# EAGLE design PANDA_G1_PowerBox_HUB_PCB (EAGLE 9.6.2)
BOARD_NAME: PwrBoxHUB

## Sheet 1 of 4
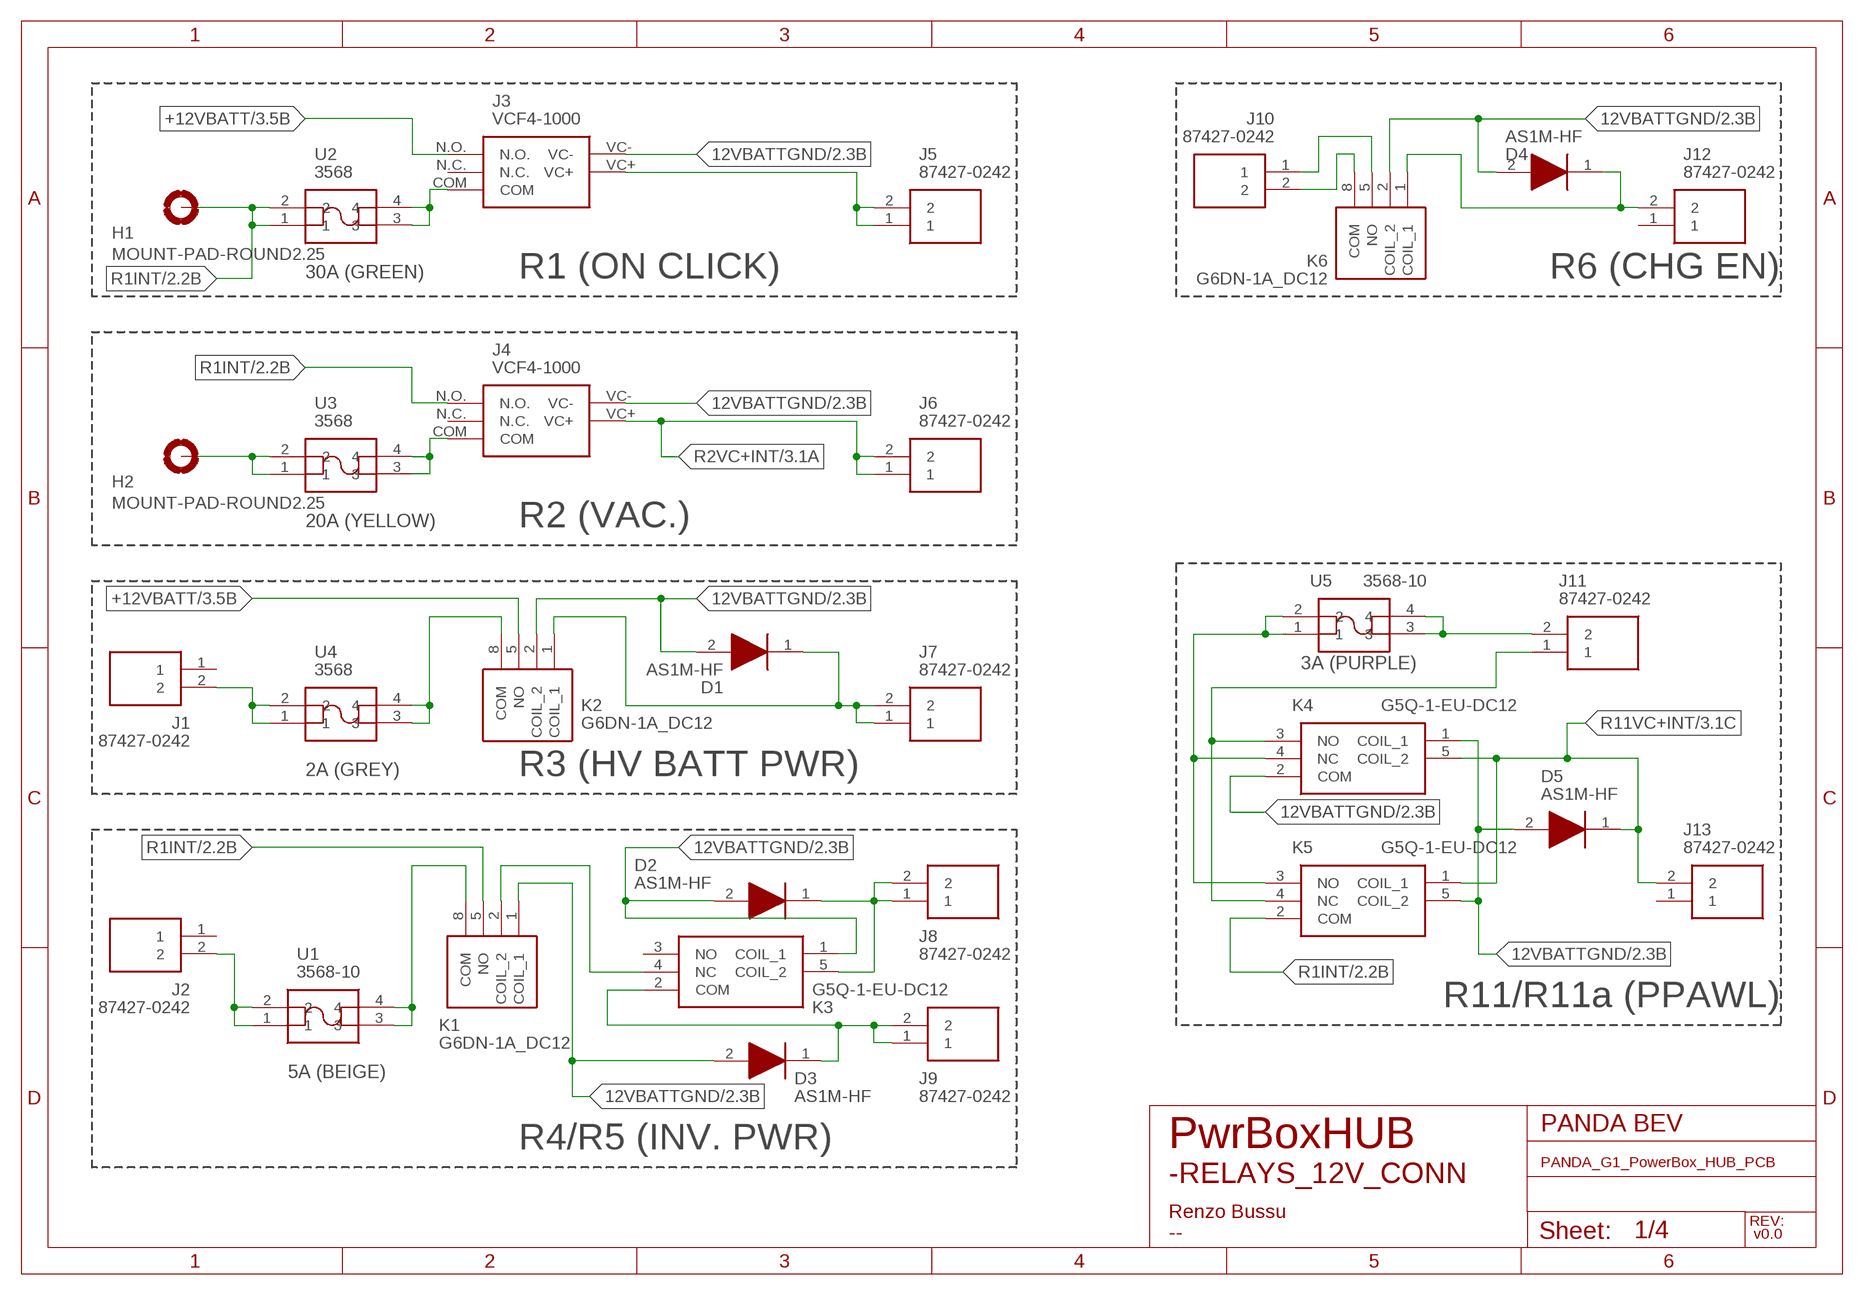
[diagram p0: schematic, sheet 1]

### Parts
D1  AS1M-HF  [DIOM5126X215N]
D2  AS1M-HF  [DIOM5126X215N]
D3  AS1M-HF  [DIOM5126X215N]
D4  AS1M-HF  [DIOM5126X215N]
D5  AS1M-HF  [DIOM5126X215N]
H1  MOUNT-PAD-ROUND2.25  [2,25-PAD]
H2  MOUNT-PAD-ROUND2.25  [2,25-PAD]
J1  87427-0242  [874270242]
J2  87427-0242  [874270242]
J3  VCF4-1000  [VCF4-1000]
J4  VCF4-1000  [VCF4-1000]
J5  87427-0242  [874270242]
J6  87427-0242  [874270242]
J7  87427-0242  [874270242]
J8  87427-0242  [874270242]
J9  87427-0242  [874270242]
J10  87427-0242  [874270242]
J11  87427-0242  [874270242]
J12  87427-0242  [874270242]
J13  87427-0242  [874270242]
K1  G6DN-1A_DC12  [G6DN1ADC12]
K2  G6DN-1A_DC12  [G6DN1ADC12]
K3  G5Q-1-EU-DC12  [G5Q1EUDC12]
K4  G5Q-1-EU-DC12  [G5Q1EUDC12]
K5  G5Q-1-EU-DC12  [G5Q1EUDC12]
K6  G6DN-1A_DC12  [G6DN1ADC12]
U1  3568-10  [356810]
U2  3568  [3568]
U3  3568  [3568]
U4  3568  [3568]
U5  3568-10  [356810]

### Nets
12VBATTGND: D1.2(A) D2.2(A) D3.2(A) D4.2(A) D5.2(A) J3.VC- J4.VC- K1.1(COIL_1) K2.2(COIL_2) K3.1(COIL_1) K4.1(COIL_1) K4.2(COM) K5.5(COIL_2) K6.2(COIL_2) ; also sheet 2,3,4
+12VBATT: J3.N.O. K2.5(NO) ; also sheet 3,4
N$2: J3.COM U2.3 U2.4
N$3: J4.COM U3.3 U3.4
N$4: J3.VC+ J5.1 J5.2
N$5: H2.B2,25(MOUNT) U3.1 U3.2
N$6: K2.8(COM) U4.3 U4.4
N$7: J1.2 U4.1 U4.2
N$8: D1.1(K) J7.1 J7.2 K2.1(COIL_1)
N$9: J2.2 U1.1 U1.2
N$10: K1.8(COM) U1.3 U1.4
N$11: D2.1(K) J8.1 J8.2 K3.5(COIL_2)
N$12: D3.1(K) J9.1 J9.2 K3.2(COM)
N$13: K1.2(COIL_2) K3.4(NC)
N$14: J10.2 K6.8(COM)
N$15: J10.1 K6.5(NO)
N$16: D4.1(K) J12.2 K6.1(COIL_1)
N$27: J11.2 U5.3 U5.4
N$28: K4.4(NC) K5.3(NO) U5.1 U5.2
N$30: J11.1 K4.3(NO) K5.4(NC)
R1INT: H1.B2,25(MOUNT) J4.N.O. K1.5(NO) K5.2(COM) U2.1 U2.2 ; also sheet 2,4
R2VC+INT: J4.VC+ J6.1 J6.2 ; also sheet 3
R11VC+INT: D5.1(K) J13.2 K4.5(COIL_2) K5.1(COIL_1) ; also sheet 3
Unconnected: J1.1 J2.1 J3.N.C. J4.N.C. J12.1 J13.1 K3.3(NO)

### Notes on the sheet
- 30A (GREEN) | R1 (ON CLICK) | R6 (CHG EN)
- 20A (YELLOW) | R2 (VAC.)
- 3A (PURPLE)
- 2A (GREY) | R3 (HV BATT PWR)
- R11/R11a (PPAWL)
- 5A (BEIGE)
- R4/R5 (INV. PWR)
- -RELAYS_12V_CONN
- Renzo Bussu
- v0.0
- --

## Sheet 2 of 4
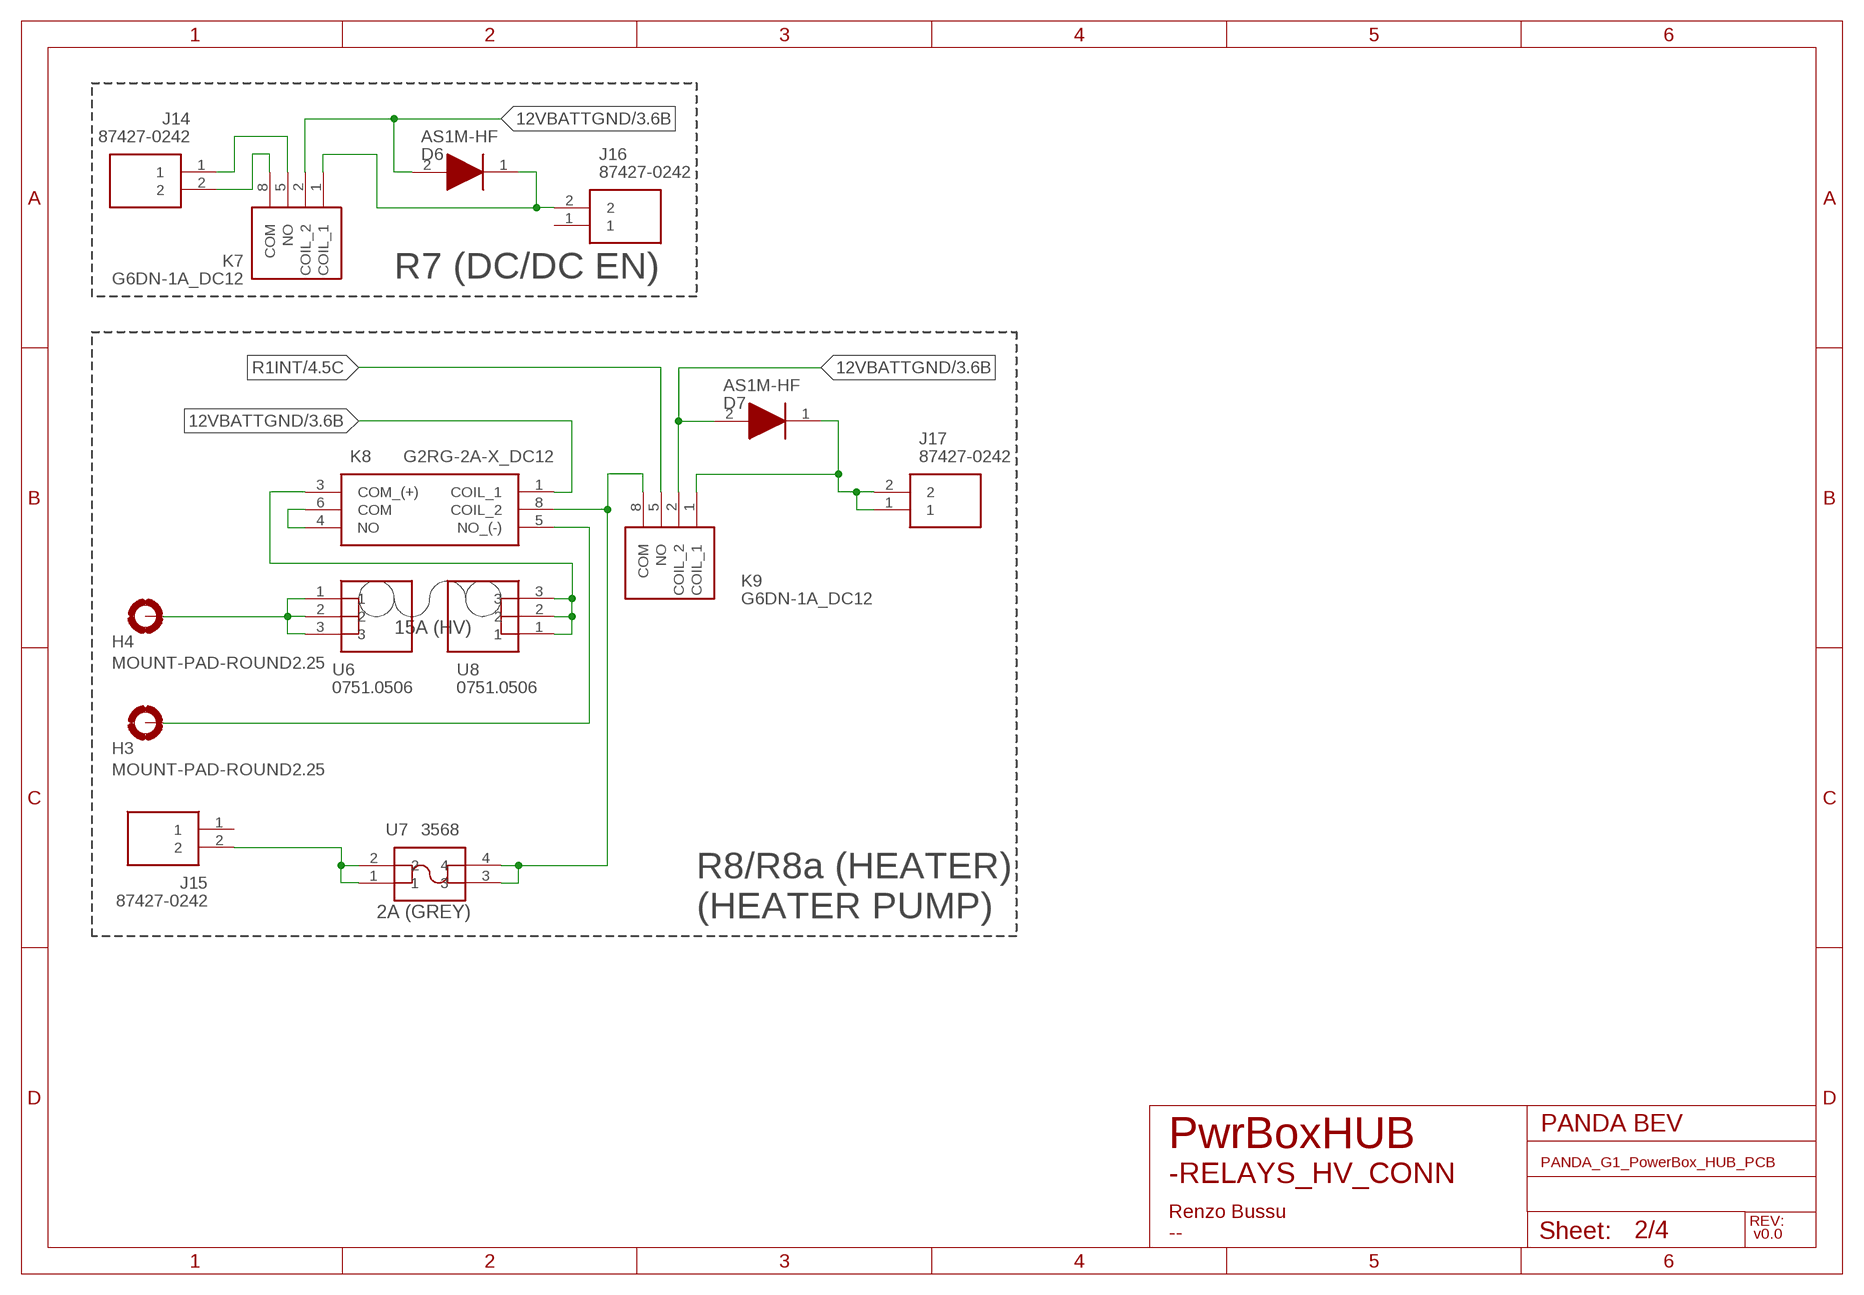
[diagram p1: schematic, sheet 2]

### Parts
D6  AS1M-HF  [DIOM5126X215N]
D7  AS1M-HF  [DIOM5126X215N]
H3  MOUNT-PAD-ROUND2.25  [2,25-PAD]
H4  MOUNT-PAD-ROUND2.25  [2,25-PAD]
J14  87427-0242  [874270242]
J15  87427-0242  [874270242]
J16  87427-0242  [874270242]
J17  87427-0242  [874270242]
K7  G6DN-1A_DC12  [G6DN1ADC12]
K8  G2RG-2A-X_DC12  [G2RG2AXDC12]
K9  G6DN-1A_DC12  [G6DN1ADC12]
U6  0751.0506  [07510506]
U7  3568  [3568]
U8  0751.0506  [07510506]

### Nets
12VBATTGND: D6.2(A) D7.2(A) K7.2(COIL_2) K8.1(COIL_1) K9.2(COIL_2) ; also sheet 1,3,4
N$17: J14.2 K7.8(COM)
N$18: J14.1 K7.5(NO)
N$19: D6.1(K) J16.2 K7.1(COIL_1)
N$20: H3.B2,25(MOUNT) K8.5(NO_(-))
N$21: K8.4(NO) K8.6(COM)
N$22: K8.3(COM_(+)) U8.1 U8.2 U8.3
N$23: D7.1(K) J17.1 J17.2 K9.1(COIL_1)
N$24: H4.B2,25(MOUNT) U6.1 U6.2 U6.3
N$25: K8.8(COIL_2) K9.8(COM) U7.3 U7.4
N$26: J15.2 U7.1 U7.2
R1INT: K9.5(NO) ; also sheet 1,4
Unconnected: J15.1 J16.1

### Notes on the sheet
- R7 (DC/DC EN)
- 15A (HV)
- 2A (GREY)
- R8/R8a (HEATER)
  (HEATER PUMP)
- -RELAYS_HV_CONN
- Renzo Bussu
- v0.0
- --

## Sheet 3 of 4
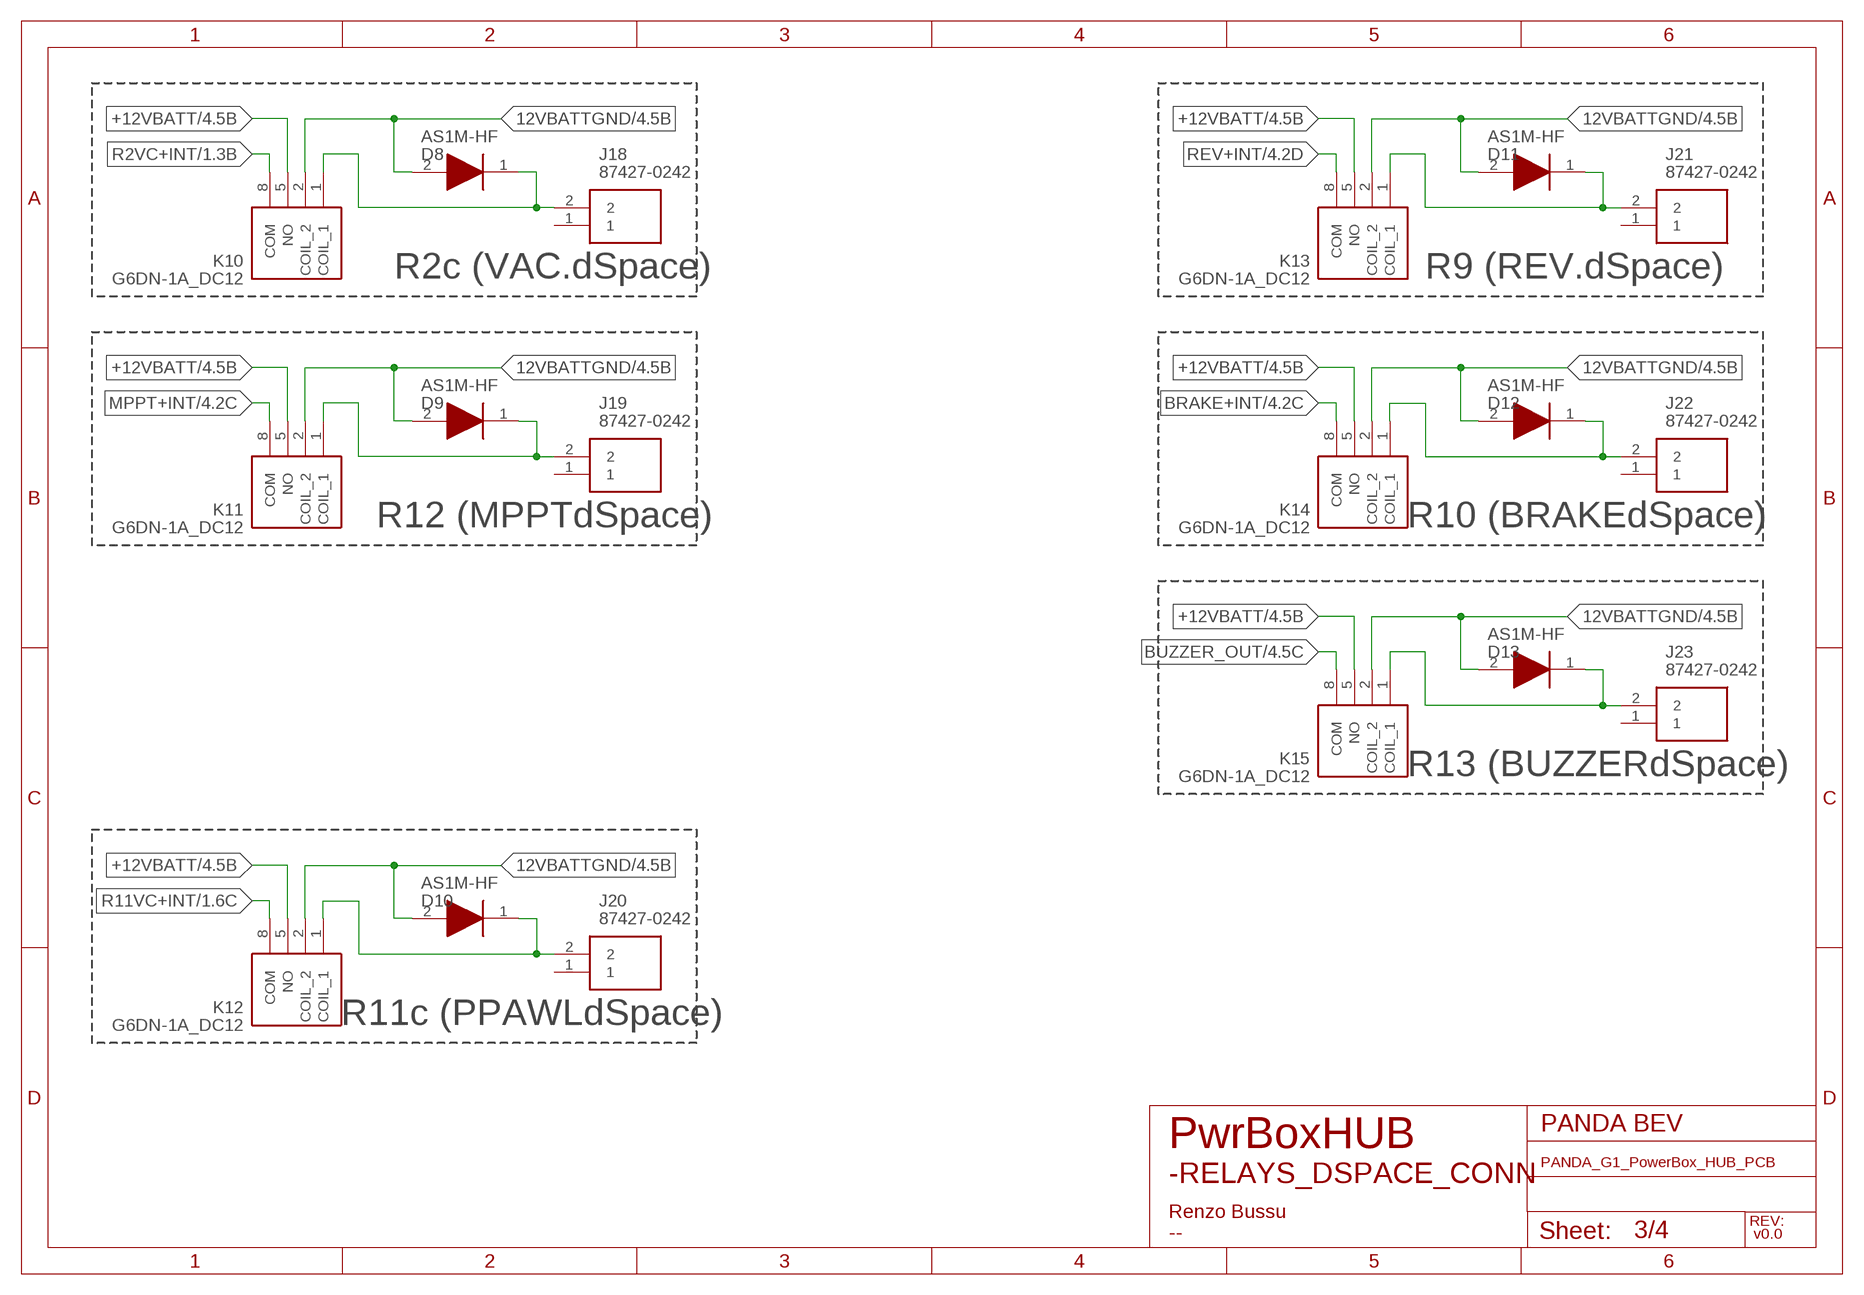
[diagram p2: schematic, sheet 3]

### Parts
D8  AS1M-HF  [DIOM5126X215N]
D9  AS1M-HF  [DIOM5126X215N]
D10  AS1M-HF  [DIOM5126X215N]
D11  AS1M-HF  [DIOM5126X215N]
D12  AS1M-HF  [DIOM5126X215N]
D13  AS1M-HF  [DIOM5126X215N]
J18  87427-0242  [874270242]
J19  87427-0242  [874270242]
J20  87427-0242  [874270242]
J21  87427-0242  [874270242]
J22  87427-0242  [874270242]
J23  87427-0242  [874270242]
K10  G6DN-1A_DC12  [G6DN1ADC12]
K11  G6DN-1A_DC12  [G6DN1ADC12]
K12  G6DN-1A_DC12  [G6DN1ADC12]
K13  G6DN-1A_DC12  [G6DN1ADC12]
K14  G6DN-1A_DC12  [G6DN1ADC12]
K15  G6DN-1A_DC12  [G6DN1ADC12]

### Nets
12VBATTGND: D8.2(A) D9.2(A) D10.2(A) D11.2(A) D12.2(A) D13.2(A) K10.2(COIL_2) K11.2(COIL_2) K12.2(COIL_2) K13.2(COIL_2) K14.2(COIL_2) K15.2(COIL_2) ; also sheet 1,2,4
+12VBATT: K10.5(NO) K11.5(NO) K12.5(NO) K13.5(NO) K14.5(NO) K15.5(NO) ; also sheet 1,4
BRAKE+INT: K14.8(COM) ; also sheet 4
BUZZER_OUT: K15.8(COM) ; also sheet 4
MPPT+INT: K11.8(COM) ; also sheet 4
N$32: D8.1(K) J18.2 K10.1(COIL_1)
N$33: D10.1(K) J20.2 K12.1(COIL_1)
N$36: D11.1(K) J21.2 K13.1(COIL_1)
N$37: D12.1(K) J22.2 K14.1(COIL_1)
N$38: D13.1(K) J23.2 K15.1(COIL_1)
N$39: D9.1(K) J19.2 K11.1(COIL_1)
R2VC+INT: K10.8(COM) ; also sheet 1
R11VC+INT: K12.8(COM) ; also sheet 1
REV+INT: K13.8(COM) ; also sheet 4
Unconnected: J18.1 J19.1 J20.1 J21.1 J22.1 J23.1

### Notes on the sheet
- R2c (VAC.dSpace) | R9 (REV.dSpace)
- R12 (MPPTdSpace) | R10 (BRAKEdSpace)
- R13 (BUZZERdSpace)
- R11c (PPAWLdSpace)
- -RELAYS_DSPACE_CONN
- Renzo Bussu
- v0.0
- --

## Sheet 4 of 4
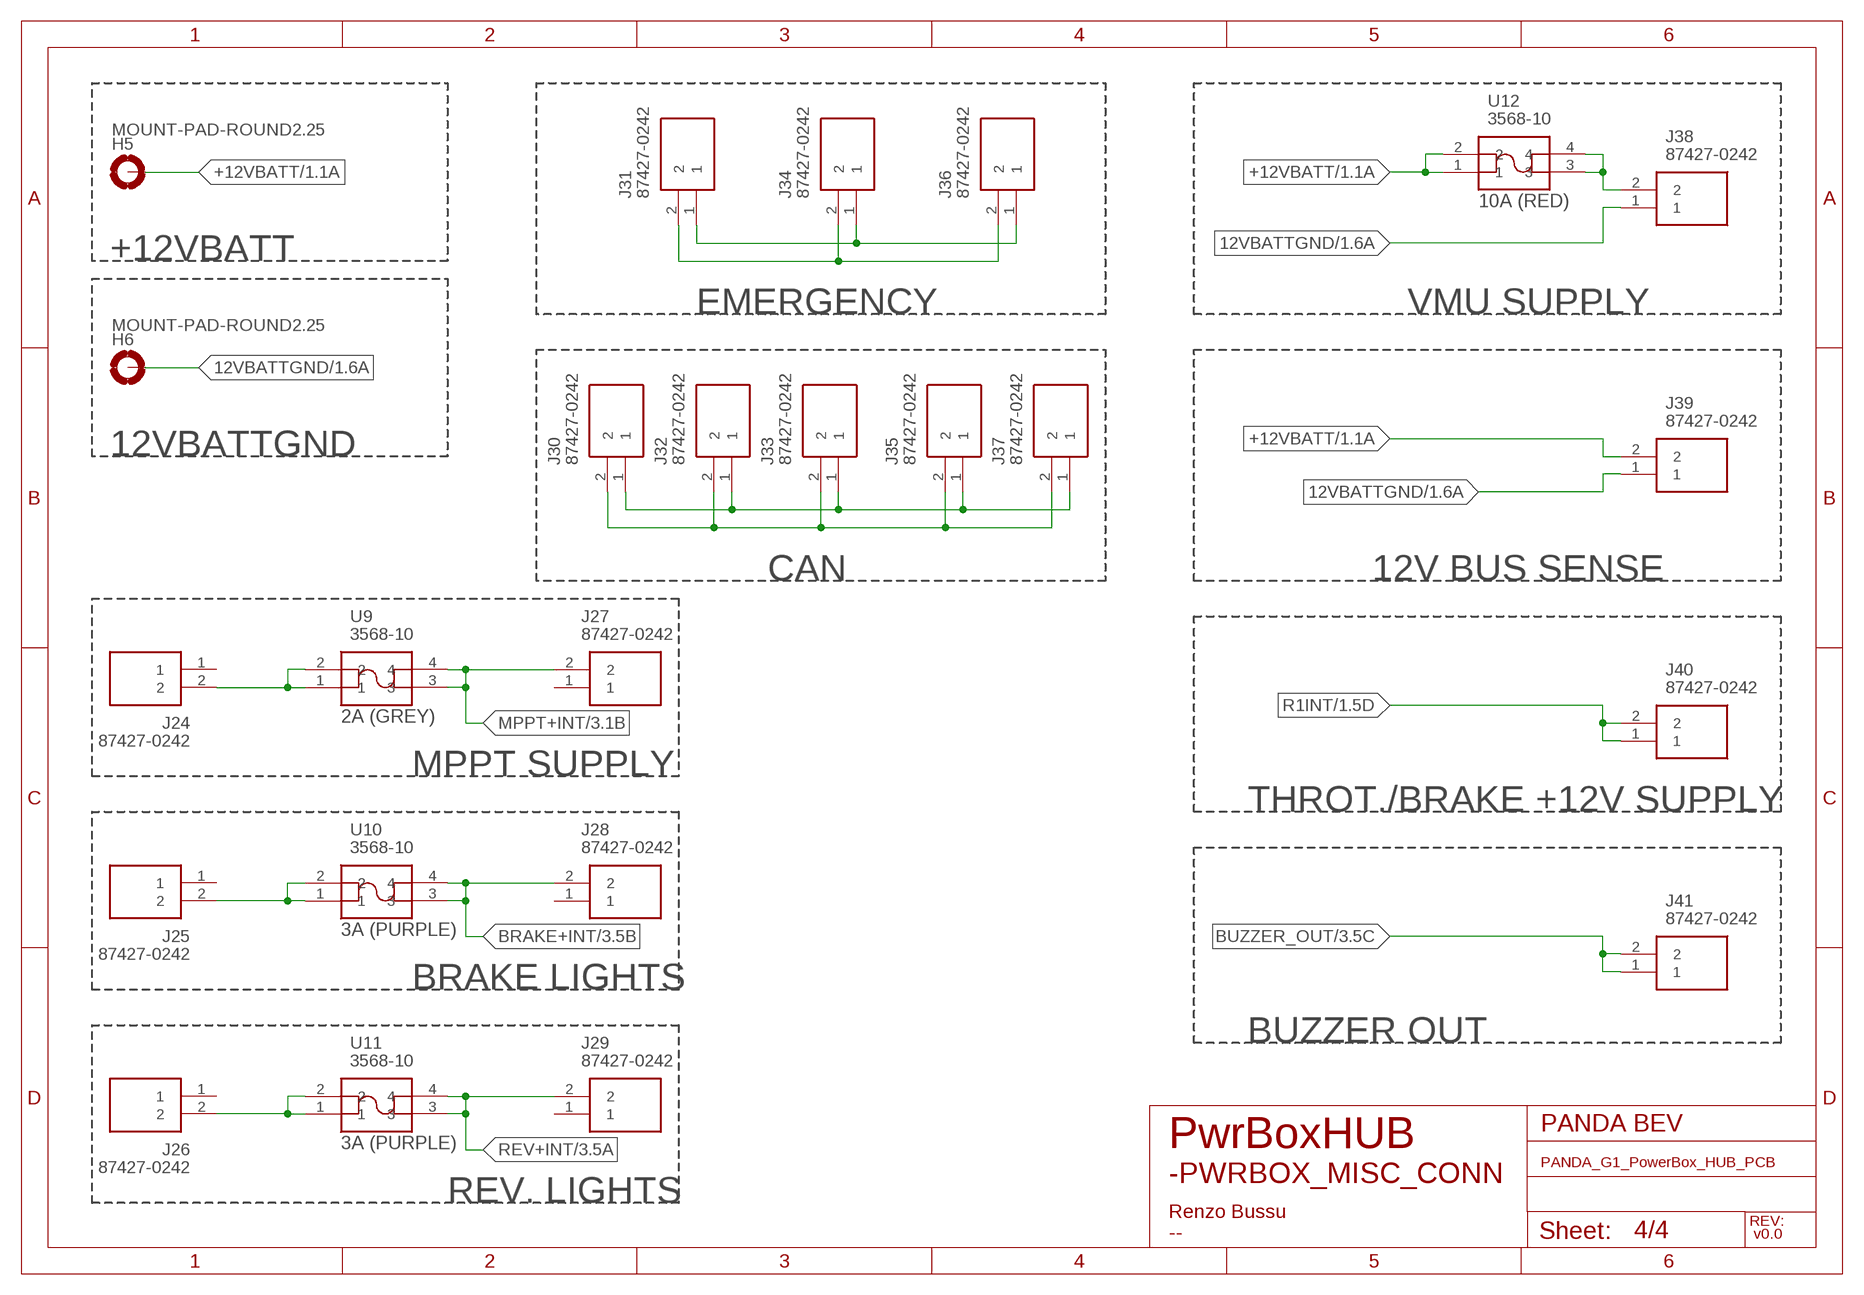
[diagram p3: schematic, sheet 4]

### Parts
H5  MOUNT-PAD-ROUND2.25  [2,25-PAD]
H6  MOUNT-PAD-ROUND2.25  [2,25-PAD]
J24  87427-0242  [874270242]
J25  87427-0242  [874270242]
J26  87427-0242  [874270242]
J27  87427-0242  [874270242]
J28  87427-0242  [874270242]
J29  87427-0242  [874270242]
J30  87427-0242  [874270242]
J31  87427-0242  [874270242]
J32  87427-0242  [874270242]
J33  87427-0242  [874270242]
J34  87427-0242  [874270242]
J35  87427-0242  [874270242]
J36  87427-0242  [874270242]
J37  87427-0242  [874270242]
J38  87427-0242  [874270242]
J39  87427-0242  [874270242]
J40  87427-0242  [874270242]
J41  87427-0242  [874270242]
U9  3568-10  [356810]
U10  3568-10  [356810]
U11  3568-10  [356810]
U12  3568-10  [356810]

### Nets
12VBATTGND: H6.B2,25(MOUNT) J38.1 J39.1 ; also sheet 1,2,3
+12VBATT: H5.B2,25(MOUNT) J39.2 U12.1 U12.2 ; also sheet 1,3
BRAKE+INT: J28.2 U10.3 U10.4 ; also sheet 3
BUZZER_OUT: J41.1 J41.2 ; also sheet 3
CAN_N [CAN diff]: J30.1 J32.1 J33.1 J35.1 J37.1
CAN_P [CAN diff]: J30.2 J32.2 J33.2 J35.2 J37.2
MPPT+INT: J27.2 U9.3 U9.4 ; also sheet 3
N$1: J38.2 U12.3 U12.4
N$29: J25.2 U10.1 U10.2
N$31: J24.2 U9.1 U9.2
N$34: J31.2 J34.2 J36.2
N$35: J26.2 U11.1 U11.2
N$40: J31.1 J34.1 J36.1
R1INT: J40.1 J40.2 ; also sheet 1,2
REV+INT: J29.2 U11.3 U11.4 ; also sheet 3
Unconnected: J24.1 J25.1 J26.1 J27.1 J28.1 J29.1

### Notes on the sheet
- 10A (RED)
- EMERGENCY | VMU SUPPLY
- CAN | 12V BUS SENSE
- 2A (GREY)
- MPPT SUPPLY
- THROT./BRAKE +12V SUPPLY
- 3A (PURPLE)
- BRAKE LIGHTS
- BUZZER OUT
- 3A (PURPLE)
- -PWRBOX_MISC_CONN
- REV. LIGHTS
- Renzo Bussu
- v0.0
- --

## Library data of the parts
D1-D13 = AS1M-HF:AS1M-HF: Rectifiers AUTOMOTIVE RECTIFIER GEN PURP 1000V 1A SMA SMD General Purpose Rectifiers; DESCRIPTION: Rectifiers AUTOMOTIVE RECTIFIER GEN PURP 1000V 1A SMA SMD General Purpose Rectifiers; HEIGHT: 2.15mm; MANUFACTURER_NAME: Comchip Technology; MANUFACTURER_PART_NUMBER: AS1M-HF
H1-H6 = EVERGRIN_holes:MOUNT-PAD-ROUND: MOUNTING PAD, round
J1 J2 J5-J41 = 87427-0242:87427-0242: Headers & Wire Housings MINI-FIT JR. W-TO-B; ALLIED_NUMBER: 70374145; DESCRIPTION: Headers & Wire Housings MINI-FIT JR. W-TO-B; HEIGHT: 13.7mm; MANUFACTURER_NAME: Molex; MANUFACTURER_PART_NUMBER: 87427-0242; RS_PART_NUMBER: 6705887P; RS_PRICE-STOCK: http://uk.rs-online.com/web/p/products/6705887P
J3 J4 = VCF4-1000:VCF4-1000: Relay Socket; PCB; VTF Series; 1 Pole; Quick-Connect; w/o Grounding Provision Source: Datasheet; ALLIED_NUMBER: 70198724; DESCRIPTION: Relay Socket; PCB; VTF Series; 1 Pole; Quick-Connect; w/o Grounding Provision; HEIGHT: mm; MANUFACTURER_NAME: TE Connectivity; MANUFACTURER_PART_NUMBER: VCF4-1000; RS_PART_NUMBER: 2509255350; RS_PRICE-STOCK: http://uk.rs-online.com/web/p/products/2509255350
K1 K2 K6 K7 K9-K15 = G6DN-1A_DC12:G6DN-1A_DC12: General Purpose Relays Source: Datasheet; ALLIED_NUMBER: 70788813; DESCRIPTION: General Purpose Relays; HEIGHT: 12.5mm; MANUFACTURER_NAME: Omron Electronics; MANUFACTURER_PART_NUMBER: G6DN-1A DC12; RS_PART_NUMBER: 2051950; RS_PRICE-STOCK: http://uk.rs-online.com/web/p/products/2051950
K3-K5 = G5Q-1-EU-DC12:G5Q-1-EU-DC12: Power Relay 12VDC 5(NO)/3(NC)DC/10(NO)/3(NC)AAC SPDT (20.3mm 10.3mm 15.8mm) THT Source: Datasheet; DESCRIPTION: Power Relay 12VDC 5(NO)/3(NC)DC/10(NO)/3(NC)AAC SPDT (20.3mm 10.3mm 15.8mm) THT; HEIGHT: 16.2mm; MANUFACTURER_NAME: Omron Electronics; MANUFACTURER_PART_NUMBER: G5Q-1-EU-DC12
K8 = G2RG-2A-X_DC12:G2RG-2A-X_DC12: General Purpose Relays 500VDC/10A high-voltage switching relay (2-pole wiring) Source: Datasheet; DESCRIPTION: General Purpose Relays 500VDC/10A high-voltage switching relay (2-pole wiring); HEIGHT: 29.5mm; MANUFACTURER_NAME: Omron Electronics; MANUFACTURER_PART_NUMBER: G2RG-2A-X DC12
U1 U5 U9-U12 = 3568-10:3568-10: FUSE SOCKET (RED) / BULK Source: Datasheet; ALLIED_NUMBER: 71172303; DESCRIPTION: FUSE SOCKET (RED) / BULK; HEIGHT: 7.5mm; MANUFACTURER_NAME: Keystone Electronics; MANUFACTURER_PART_NUMBER: 3568-10
U2-U4 U7 = 3568:3568: Fuse Holder 30A 500V 1 Circuit Blade Through Hole Source: Datasheet; DESCRIPTION: Fuse Holder 30A 500V 1 Circuit Blade Through Hole; HEIGHT: 7.5mm; MANUFACTURER_NAME: Keystone Electronics; MANUFACTURER_PART_NUMBER: 3568
U6 U8 = 0751.0506:0751.0506: Schurter 0751 Copper Alloy PCB Mount Fuse Clip for 10.3 x 85mm Source: Datasheet; ALLIED_NUMBER: 70255345; DESCRIPTION: Schurter 0751 Copper Alloy PCB Mount Fuse Clip for 10.3 x 85mm; HEIGHT: 20.7mm; MANUFACTURER_NAME: SCHURTER; MANUFACTURER_PART_NUMBER: 0751.0506; RS_PART_NUMBER: 8936991; RS_PRICE-STOCK: http://uk.rs-online.com/web/p/products/8936991

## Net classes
0 default: width 0.254 mm, clearance 0.254 mm
1 CAN diff: width 1.219 mm, clearance 1 mm to class 0, clearance 1 mm

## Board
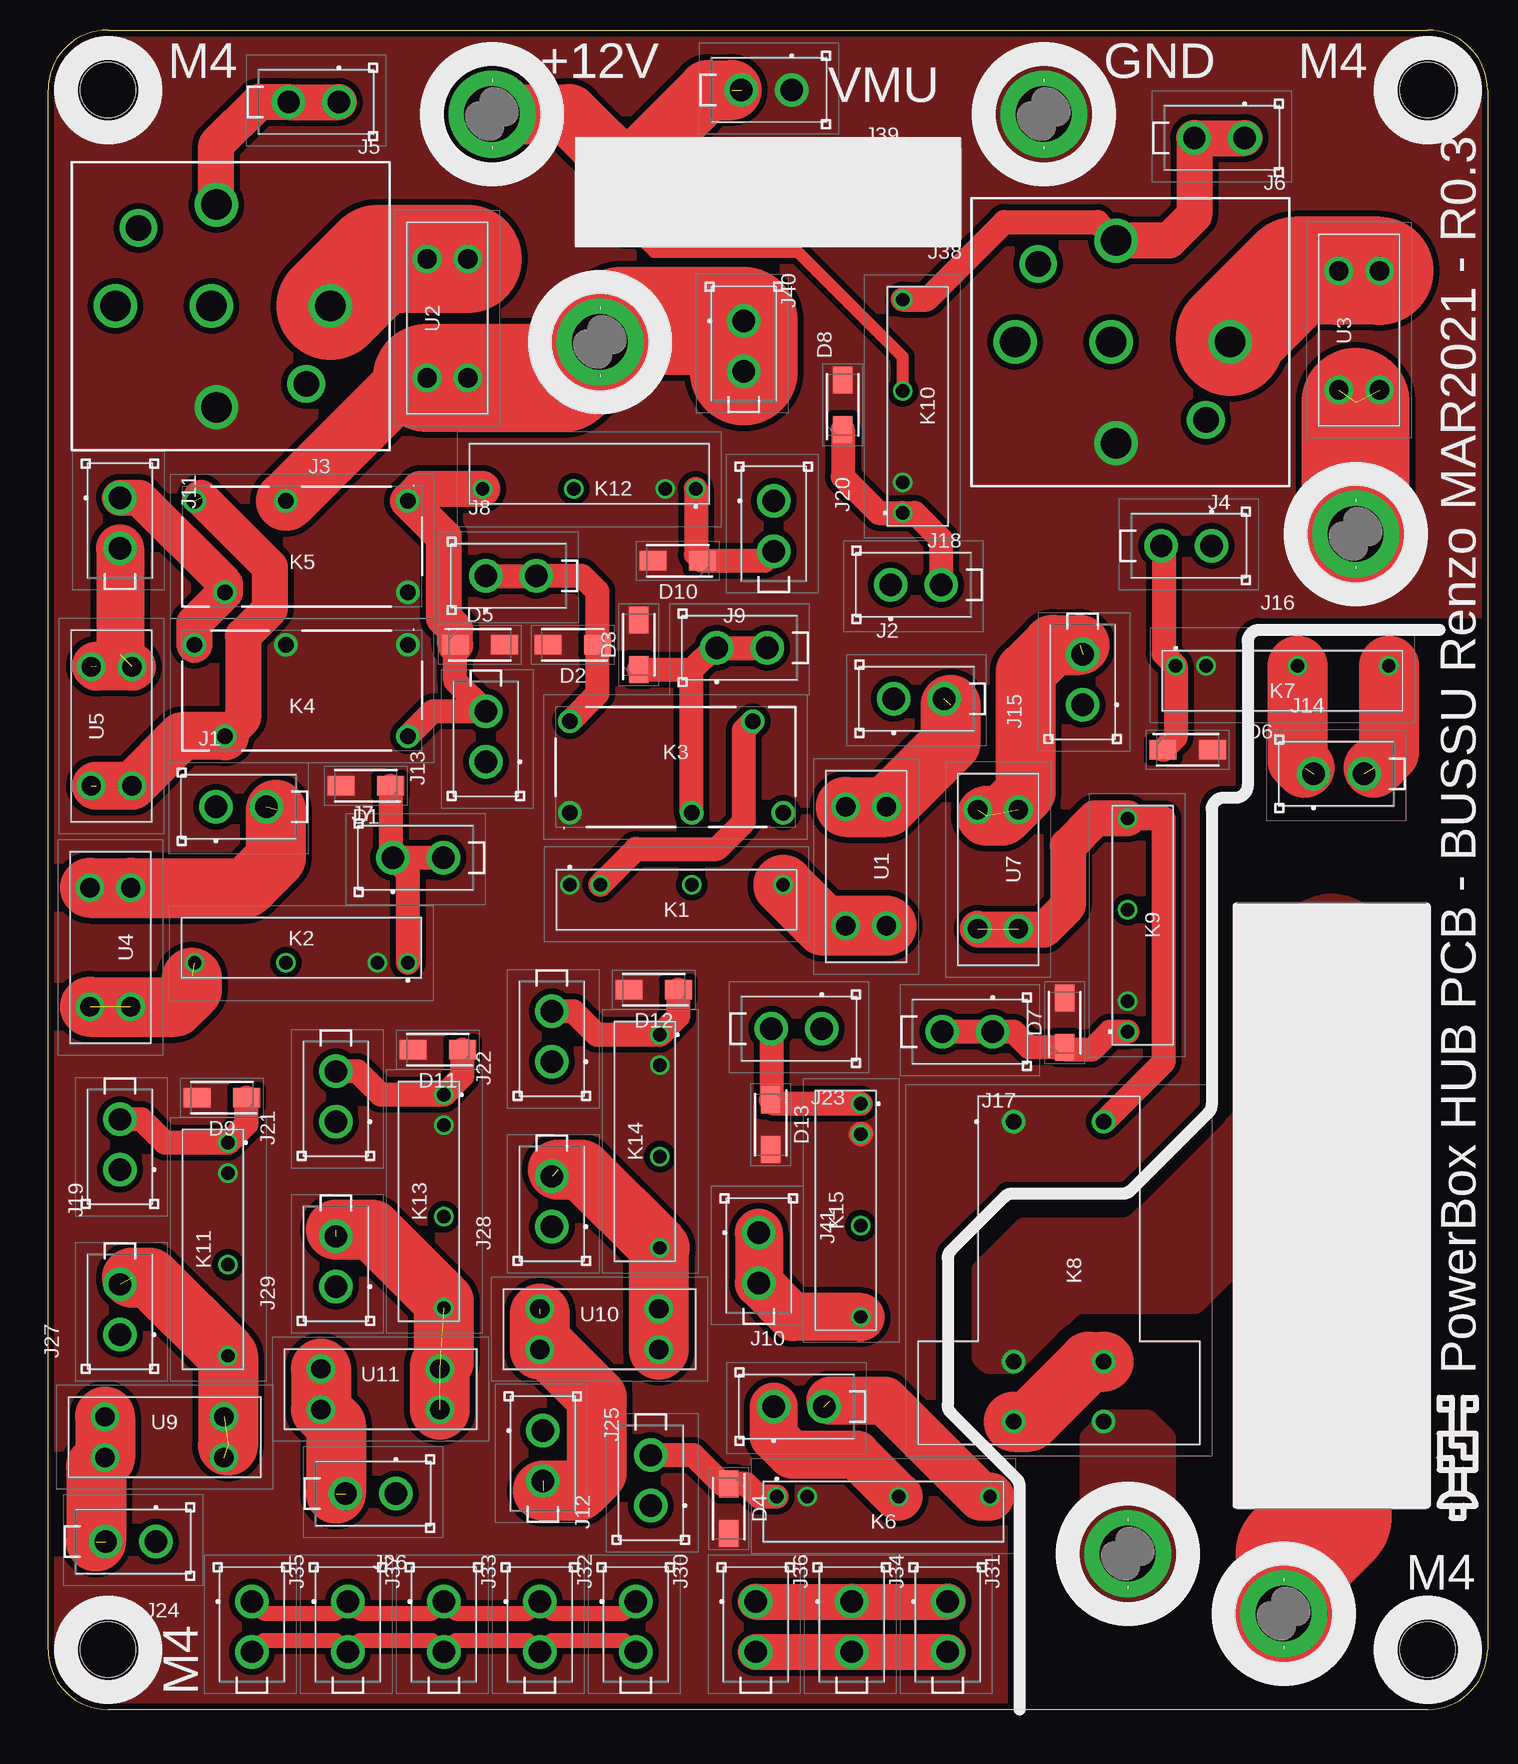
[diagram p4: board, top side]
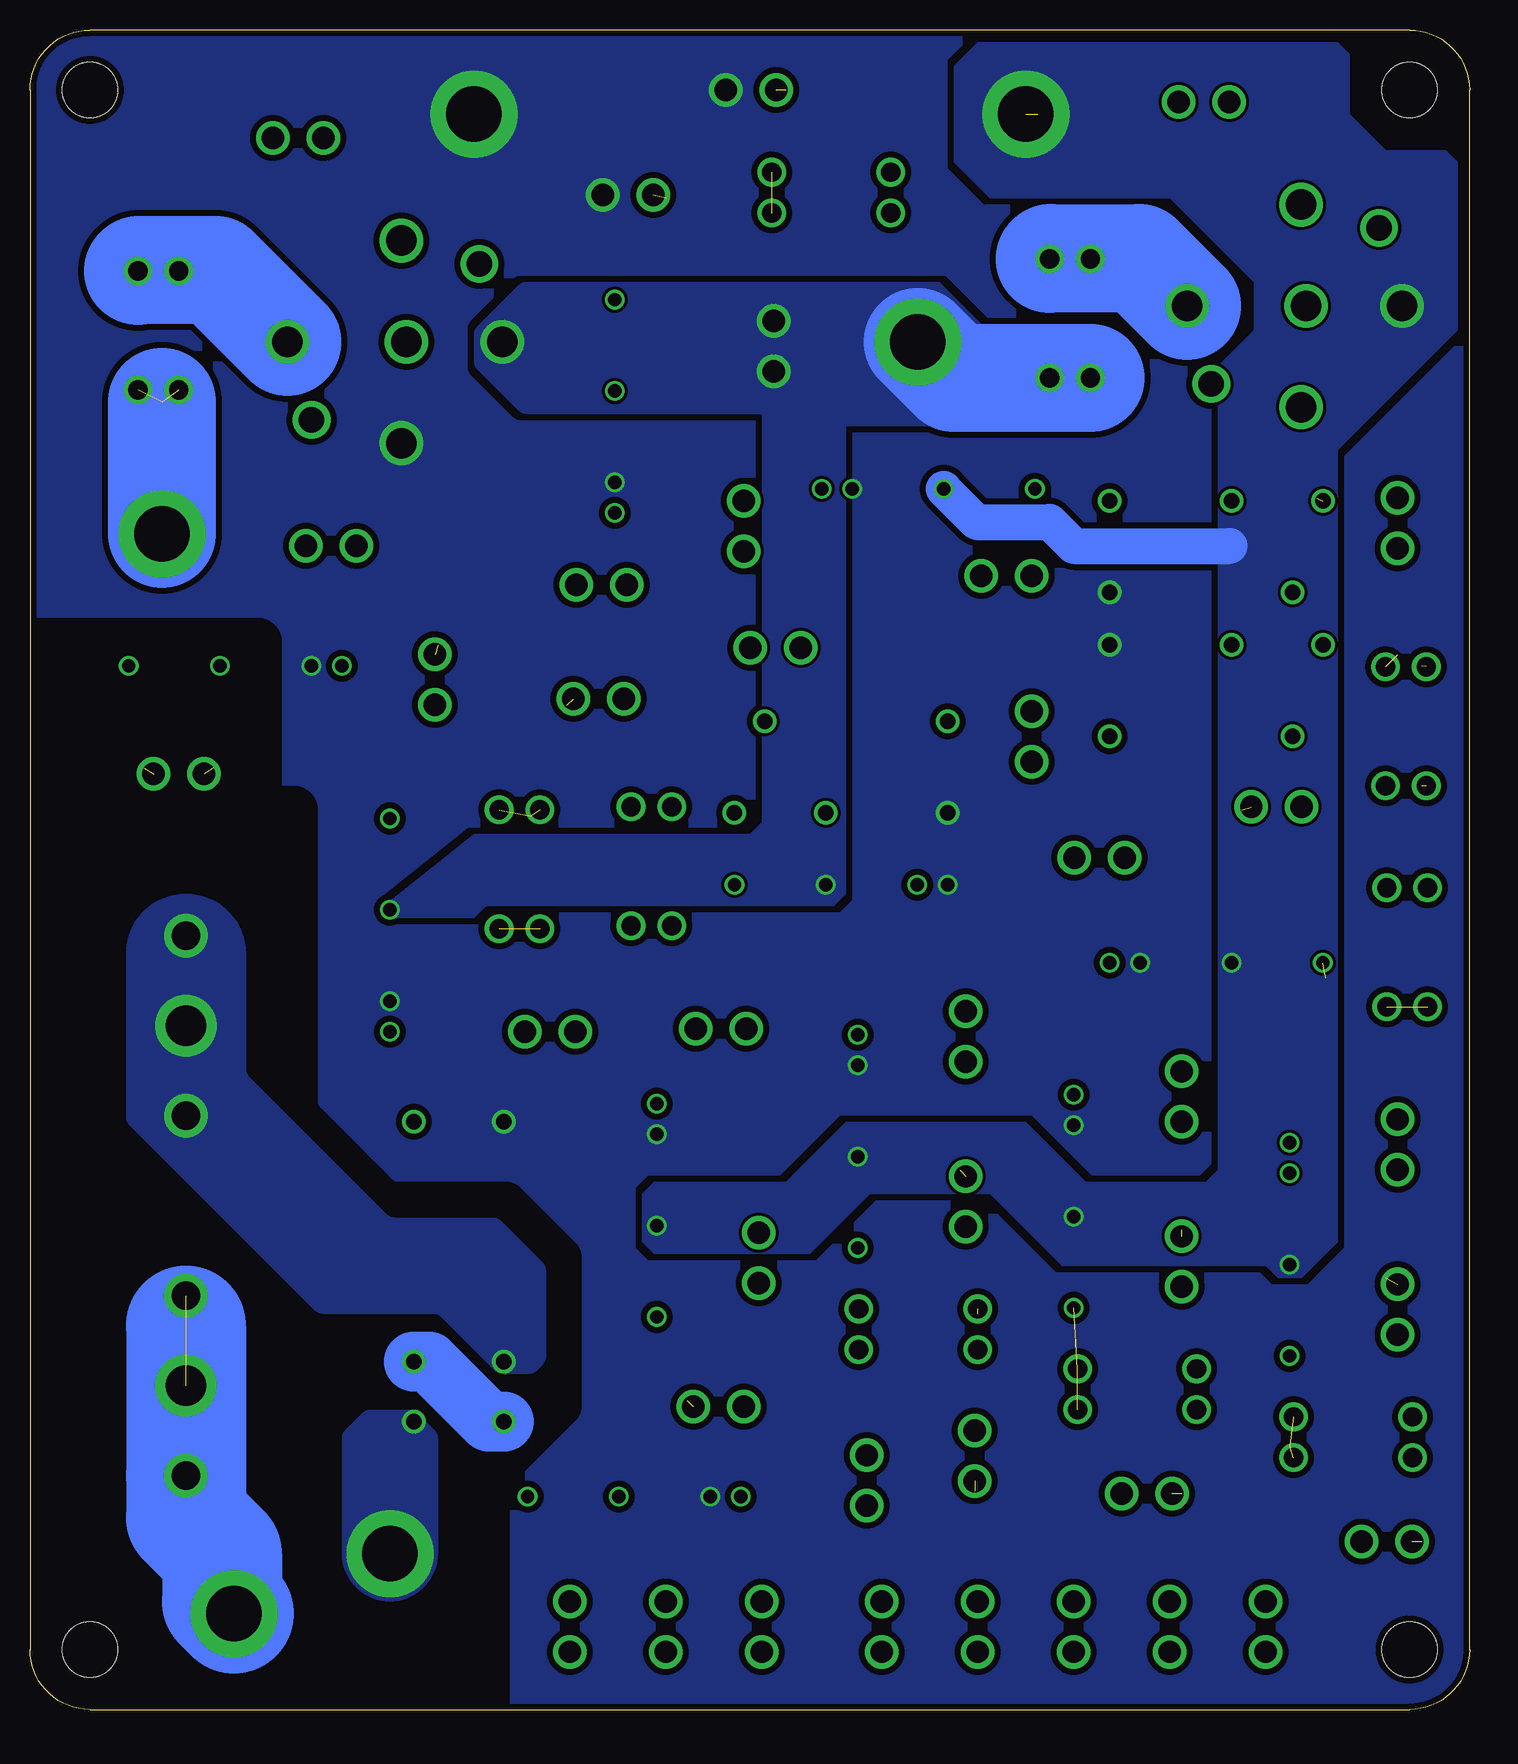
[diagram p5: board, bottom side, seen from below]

Size 120 x 140 mm. Coordinates in mm from the lower left corner, seen from the top.
Outline: 0,5 0,135 arc-90 5,140 115,140 arc-90 120,135 120,5 arc-90 115,0 5,0 arc-90 0,5
Copper layers (1*16): Top 0.035mm / dielectric 1.5mm / Bottom 0.035mm
Design rules "EVERGRIN_MDSRL": minimum track width 8mil, minimum drill 8mil, track to track 8mil, track to pad 8mil, pad to pad 8mil, via to via 8mil, smd to smd 0mil, copper to edge 10mil, drill to drill 10mil, minimum pad ring 8mil, minimum via ring 8mil, stop-mask expansion 4mil, vias tented up to drill 0mil, thermal gap 10mil
Holes 4.6 mm at 5,5 115,5 5,135 115,135
tRestrict: 18 lines
bRestrict: 19 lines

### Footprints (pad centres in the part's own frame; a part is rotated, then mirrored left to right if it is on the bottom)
DIOM5126X215N = smd 2.25 x 1.6: 1 -2.05,0; 2 2.05,0
2,25-PAD = drill 4.6 pad 7.25: B2,25 0,0
874270242 = drill 1.85 pad 2.775: 1 0,0; 2 0,4.2
VCF4-1000 = drill 2.537 pad 3.65: COM -21.539,0; N.C. -11.633,0; N.O. -3.632,0; VC+ -12.04,-8.445; VC- -12.04,8.445 | drill 2.108 pad 3.15: MECH1 -19.533,6.502; MECH2 -5.537,-6.502
G6DN1ADC12 = drill 1.1 pad 1.65: 1 0,0; 2 2.54,0; 5 10.16,0; 8 17.78,0
G5Q1EUDC12 = drill 1.3 pad 1.95: 1 0,0; 2 10.16,0; 3 17.78,0; 4 15.24,7.62; 5 0,7.62
G2RG2AXDC12 = drill 1.3 pad 1.95: 1 0,0; 3 20,0; 4 25,0; 5 25,7.5; 6 20,7.5; 8 0,7.5
356810 = drill 1.6 pad 2.4: 1 0,0; 2 0,3.4; 3 9.92,0; 4 9.92,3.4
3568 = drill 1.6 pad 2.4: 1 0,0; 2 0,3.4; 3 9.92,0; 4 9.92,3.4
07510506 = drill 2.4 pad 3.6: 1 -7.493,0; 3 7.493,0 | drill 3.4 pad 5.1: 2 0,0

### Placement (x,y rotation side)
D1  26.5,77 180 top
D2  43.75,88.75 180 top
D3  49.25,88.75 90 top
D4  56.75,16.75 270 top
D5  36,88.75 0 top
D6  95,80 0 top
D7  84.75,57.25 90 top
D8  66.25,108.75 90 top
D9  14.5,51 180 top
D10  52.5,95.75 180 top
D11  32.5,55 180 top
D12  50.5,60 180 top
D13  60.25,48.75 270 top
H1  46,114 0 top
H2  109,98 0 top
H3  90,13 0 top
H4  103,8 0 top
H5  37,133 0 top
H6  83,133 0 top
J1  14,75.25 270 top
J2  70.5,84.25 270 top
J3  2,117 180 top
J4  77,114 180 top
J5  24.25,134 90 top
J6  99.75,131 90 top
J7  28.75,71 270 top
J8  36.5,94.5 270 top
J9  55.75,88.5 270 top
J10  60.5,25.25 270 top
J11  6,101 180 top
J12  50.25,17 0 top
J13  36.5,79 0 top
J14  105.5,78 270 top
J15  86.25,83.75 0 top
J16  97,97 90 top
J17  78.75,56.5 90 top
J18  70.25,93.75 270 top
J19  6,45 0 top
J20  60.5,100.75 180 top
J21  24,49 0 top
J22  42,54 0 top
J23  64.5,56.75 90 top
J24  9,14 90 top
J25  41.25,23.25 180 top
J26  29,18 90 top
J27  6,31.25 0 top
J28  42,40.25 0 top
J29  24,35.25 0 top
J30  49,9 180 top
J31  75,9 180 top
J32  41,9 180 top
J33  33,9 180 top
J34  67,9 180 top
J35  17,9 180 top
J36  59,9 180 top
J37  25,9 180 top
J38  72.25,126.25 90 top
J39  62,135 90 top
J40  58,115.75 180 top
J41  59.25,39.75 180 top
K1  43.5,68.75 0 top
K2  30,62.25 180 top
K3  43.5,74.75 0 top
K4  30,88.75 180 top
K5  30,100.75 180 top
K6  60.75,17.75 0 top
K7  94,87 0 top
K8  80.5,49 270 top
K9  90,56.5 90 top
K10  71.25,99.75 90 top
K11  15,47.25 270 top
K12  54,101.75 180 top
K13  33,51.25 270 top
K14  51,56.25 270 top
K15  67.75,50.5 270 top
U1  66.5,75.25 270 top
U2  35,111 90 top
U3  111,110 90 top
U4  3.5,68.5 270 top
U5  7,77 90 top
U6  107,27 270 top
U7  77.5,75 270 top
U8  107,57 90 top
U9  4.75,21 0 top
U10  41,30 0 top
U11  22.75,25 0 top
U12  48.25,124.75 0 top

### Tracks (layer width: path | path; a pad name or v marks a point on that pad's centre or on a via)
12VBATTGND
  Top 2: K15.2 67.79,48
  pour Top (isolate 0.5, rank 6, no thermals): -6,148 144,148 144,-6 -6,-6
  pour Bottom (isolate 0.5, rank 6, no thermals): -7,149 141,149 141,-7 -7,-7
+12VBATT  (2 unrouted)
  Top 1: K10.5 71.25,112.75 62.5,121.5 50.5,121.5 48.25,123.75 U12.1
  Top 5: U12.1 U12.2 | U12.2 48.25,128.25 55,135 57,135 | U12.2 43.4,133 36,133
  Bottom 3: K12.5 41.09,99 35,99 33,97 20,97
  pour Bottom (no thermals): 50,43 55,38 68,38 69,39 69,43 68,44 57,44 52,49 37,49 32,44 22,44 21,45 21,112 18,115 18,119 25,126 40,126 43,129 43,137 41,139 11,139 10,138 10,133 7,130 2,130 1,129 1,115 11,105 11,39 14,36 16,36 17,37 34,37 40,43
BRAKE+INT  (1 unrouted)
  Top 5: U10.3 U10.4 50.92,38.39 K14.8 44.47,45 42.5,45
BUZZER_OUT
  Top 4: K15.8 62.08,32.72 J41.2 J41.1
CAN_N
  Top 1.27: J35.1 17.96,8.04 24.04,8.04 J37.1 25.96,8.04 32.03,8.04 J33.1 33.97,8.04 40.03,8.04 J32.1 41.97,8.04 48.03,8.04 J30.1
CAN_P
  Top 1.27: J35.2 17.96,5.77 24.04,5.77 J37.2 25.96,5.77 32.03,5.77 J33.2 33.97,5.77 40.03,5.77 J32.2 41.97,5.77 48.03,5.77 J30.2
MPPT+INT  (3 unrouted)
  Top 5: 7,36 8.47,36 K11.8 15,22
N$1  (2 unrouted)
  Top 5: U12.3 59.42,126 67,126 | U12.3 58.17,128 58,128 58,124.75 U12.3
N$2
  Top 9: J3.COM 27.46,120.92 U2.4 U2.3
  Bottom 9: U2.3 34.92,121 27.54,121 J3.COM
N$3
  Top 9: U3.3 U3.4 103.92,119.92 98.54,114.54 J4.COM
  Bottom 9: J4.COM 104.54,120 110.92,120 U3.3
N$4
  Top 3: J3.VC+ 14.04,130.45 17.59,134 J5.2 J5.1
N$5  (2 unrouted)
  Top 9: H2.B2,25 109,109
  Bottom 9: H2.B2,25 109,109
N$6  (2 unrouted)
  Top 5: U4.3 10.58,58.58 12,60 12,61
N$7  (1 unrouted)
  Top 5: U4.1 U4.2 16.5,68.5 19,71 19,75
N$8
  Top 2: J7.2 J7.1 | D1.1 28.55,71.2 J7.1 | J7.1 30,69.75 K2.1
N$9  (1 unrouted)
  Top 5: U1.1 U1.2 75.25,80.6 75.25,83.75
N$10
  Top 5: U1.4 U1.3 64.67,65.33 61.28,68.72 K1.8
N$11
  Top 2: K3.5 45.8,84.67 D2.1 45.8,93.2 44.5,94.5 J8.2 J8.1
N$12
  Top 2: D3.1 53.7,86.7 | 53.7,86.7 55.5,88.5 J9.1 J9.2 | K3.2 53.66,86.66 53.7,86.7
N$13
  Top 2: K1.2 46.29,69 46.25,69 49,71.75 55.75,71.75 58,74 58,81.63 K3.4
N$14  (1 unrouted)
  Top 4: 65.2,25.75 69.75,25.75 77.75,17.75 K6.8
N$15
  Top 4: K6.5 67.41,21.25 62,21.25 60.5,22.75 J10.1
N$16
  Top 2: K6.1 59.25,17.75 58.2,18.8 D4.1 56.2,18.8 53.8,21.2 J12.2
N$17  (1 unrouted)
  Top 5: K7.8 111.78,79.78 110.5,78.5
N$18  (1 unrouted)
  Top 5: K7.5 104.16,79.09 104.75,78.5
N$19
  Top 2: D6.1 94,81.05 K7.1 93,88 93,96.8 J16.2
N$20
  pour Bottom (no thermals): 87,24 arc-90 88,25 91.59,25 arc-45 92.29,24.71 93.71,23.29 arc-45 94,22.59 94,13 arc-90 90,9 arc-90 86,13 86,22.59 arc-45 86.29,23.29
  pour Top (isolate 1, no thermals): 87,24 arc-90 88,25 91.59,25 arc-45 92.29,24.71 93.71,23.29 arc-45 94,22.59 94,13 arc-90 90,9 arc-90 86,13 86,22.59 arc-45 86.29,23.29
N$21
  Top 5: K8.6 86.75,29 81.75,24 K8.4
N$22
  pour Top (isolate 1, rank 2, no thermals): 81.29,28.29 85.71,32.71 arc-45 86.41,33 95.59,33 arc45 96.29,33.29 111.71,48.71 arc45 112,49.41 112,63 arc90 107,68 arc90 102,63 102,53.41 arc-45 101.71,52.71 90.29,41.29 arc-45 89.59,41 81.41,41 arc45 80.71,40.71 77.29,37.29 arc45 77,36.59 77,29.41 arc45 77.29,28.71 77.71,28.29 arc45 78.41,28 80.59,28 arc45
  pour Bottom (no thermals): 81.29,28.29 85.71,32.71 arc-45 86.41,33 95.59,33 arc45 96.29,33.29 111.71,48.71 arc45 112,49.41 112,63 arc90 107,68 arc90 102,63 102,53.41 arc-45 101.71,52.71 90.29,41.29 arc-45 89.59,41 81.41,41 arc45 80.71,40.71 77.29,37.29 arc45 77,36.59 77,29.41 arc45 77.29,28.71 77.71,28.29 arc45 78.41,28 80.59,28 arc45
N$23
  Top 2: K9.1 88.5,56.5 87,55 84.95,55 D7.1 81.8,55.2 80.5,56.5 J17.1 J17.2
N$24  (3 unrouted)
  Top 10: 104,13 107,16 107,32 | H4.B2,25 103,9
  Bottom 10: 107,32 U6.3 107,16 104,13 104,9 H4.B2,25
N$25  (1 unrouted)
  Top 2: K8.8 93,54 93,74.28 K9.8
  Top 3: K9.8 87.28,74.28 85,72 85,67 83,65 77.58,65 U7.3
N$26  (3 unrouted)
  Top 5: 78.25,74.5 79.5,74.5 81.5,76.5 81.5,86.5 83.75,88.75 86,88.75
N$27  (2 unrouted)
  Top 4: J11.2 6,87.92 | U5.3 4.08,86.92 4,87
N$28  (2 unrouted)
  Top 3: K4.4 16.25,82.62 16.25,89.5 18.5,91.75 18.5,95.25 12.75,101
  Top 4: K4.4 11.13,81.13 U5.1 4,77
N$29  (2 unrouted)
  Top 5: 41,33 U10.1 41.75,30 45.75,26 45.75,19.75 44.25,18.25 41.25,18.25
N$30
  Top 3: K4.3 12.22,90.59 K5.4 14.76,93.85 7.61,101 J11.1
N$31  (1 unrouted)
  Top 5: U9.2 U9.1 4,20.25 4,14
N$32
  Top 2: D8.1 66.25,102.75 69.25,99.75 K10.1 72.25,99.75 74.45,97.55 J18.2
N$33
  Top 2: K12.1 54,96.3 D10.1 59.7,95.75 J20.2
N$34
  Top 3: J36.2 J34.2 J31.2
N$35  (1 unrouted)
  Top 5: U11.2 U11.1 24,23.75 24,18
N$36
  Top 2: D11.1 34.55,52.8 K13.1 27.75,51.25 25.8,53.2 J21.2
N$37
  Top 2: D12.1 52.55,57.8 K14.1 45.75,56.25 43.8,58.2 J22.2
N$38
  Top 2: K15.1 60.55,50.5 60.3,50.75 | 60.3,50.75 D13.1 | J23.2 60.3,50.75
N$39
  Top 2: D9.1 16.55,48.8 K11.1 9.75,47.25 7.8,49.2 J19.2
N$40
  Top 3: J36.1 J34.1 J31.1
N$42
  Bottom 5: 88,29 86.75,29 81.75,24 80.5,24
R1INT
  Top 5: K5.2 30.09,111 U2.2
  Top 9: U2.2 43,111 H1.B2,25 47.75,115.75 J40.1 J40.2
  Bottom 9: U2.2 U2.1 43,111 H1.B2,25
  pour Bottom (no thermals): 82.71,115.29 79.29,118.71 arc45 78.59,119 44.17,119 39.17,114 39.17,107 52,107 52,68 53,67 82,67 83,66 90,66 90,67.4 83,73 60,73 59,74 59,108 78.59,108 arc45 79.29,108.29 82.71,111.71 arc45 83,112.41 83,114.59 arc45
R2VC+INT
  Top 2: K10.8 73.25,117.53 79.72,124 87.48,124 J4.VC+
  Top 3: J4.VC+ 93.44,122.44 95.55,124.55 J6.2 J6.1
R11VC+INT
  Top 2: D5.1 33.95,85.75 J13.2 32.07,83.2 K4.5
  Top 3: D5.1 33.95,90.05 33,91 33,97.75 K5.1 31,101.75 K12.8
REV+INT  (3 unrouted)
  Top 5: U11.3 32.67,28.67 33,29 33,34 27,40 24,40

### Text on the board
tPlace: M4 | +12V | GND | M4 | VMU | MAR2021 - R0.3 | PowerBox HUB PCB - BUSSU Renzo | M4 | M4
